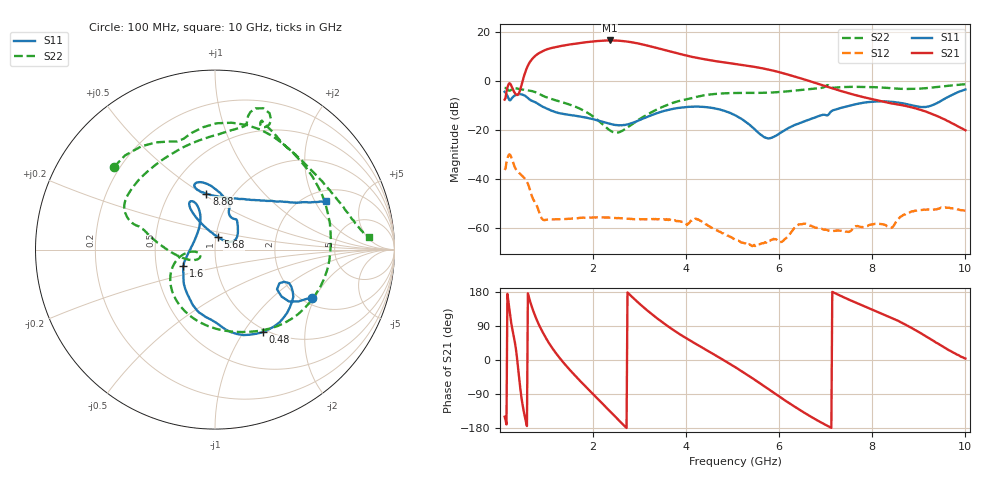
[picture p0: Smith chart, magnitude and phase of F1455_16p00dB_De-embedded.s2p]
! Integrated Device Technology
! Corporate Headquarters
! 6024 Silver Creek Valley Road
! San Jose, CA 95138  USA
! Phone:  1-408-284-8200
! Toll Free:  1-800-223-1366
! Webpage:  http://www.idt.com/
! Timing and RF Division
! 515 Groton Road, Suite 102
! Westford, MA 01886-6024
! Device:  F1455
! Description: 6-bit 0.5 dB Transmit Variable Gain Amplifier
! Frequency:  1400.0 -  2300.00 MHz
! Package:  6x6 mm Thin QFN Plastic Package: 28 pin
! State:  32
! Atten State:  16.0 dB
! Voltage:  +5.00 Volts
! Current:  217.655 mA
! Data:  The device was measured on a the F1455 evaluation board which has
!  individual transmission lines to the RF pins.  Data was collected
!  using a calibrated network analyzer.  The evaluation board was
!  de-embedded using a TRL calibration technique.
!  The reference plane is the edge of the package pin.
!  Pin  1 = CSb
!  Pin  2 = DATA
!  Pin  3 = CLK
!  Pin  4 = RSET
!  Pin  5 = GND
!  Pin  6 = RFIN  = Port 1
!  Pin  7 = GND
!  Pin  8 = NC
!  Pin  9 = NC
!  Pin 10 = NC
!  Pin 11 = NC
!  Pin 12 = NC
!  Pin 13 = NC
!  Pin 14 = /STBY
!  Pin 15 = GND
!  Pin 16 = RFOUT  = Port 2
!  Pin 17 = GND
!  Pin 18 = NC
!  Pin 19 = NC
!  Pin 20 = NC
!  Pin 21 = GND
!  Pin 22 = NC
!  Pin 23 = GND
!  Pin 24 = NC
!  Pin 25 = NC
!  Pin 26 = NC
!  Pin 27 = GND
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# GHz S dB R 50
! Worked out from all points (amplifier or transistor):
!   496 points, 100 MHz to 10 GHz, reference 50 ohm
!   highest |S21| = 16.6 dB at 2.36 GHz (marker M1)
!   |S21| within 3 dB of that: 1.129 GHz to 3.356 GHz (2.227 GHz wide, 99.3 % of centre)
!   unconditionally stable (mu >= 1): start of sweep to end of sweep
!   at 1.74 GHz: K = 45.78, MAG = 16.1 dB, |S12| = -55.8 dB
!   at 5.06 GHz: K = 250.94, MAG = 8.9 dB, |S12| = -64.8 dB
!   at 10 GHz: K = 311.19, MAG = -11.5 dB, |S12| = -52.9 dB
!   S11 on the Smith chart (normalised r, x): 100 MHz: 2.25, -1.91; 480 MHz: 0.96, -1.23; 1.6 GHz: 0.69, -0.13; 5.68 GHz: 1.02, +0.14; 8.88 GHz: 0.75, +0.52; 10 GHz: 2.48, +2.47
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0.1  -4.35 -26.3  -7.54 -149.7  -36.29 46.5  -2.77 140.7
0.26  -6.85 -24.3  -2.57 85.2  -32.06 -76.5  -3.29 95.6
0.48  -5.48 -59.8  -0.37 -113.8  -38.74 -146.9  -3.44 31.8
0.68  -7.99 -91.2  8.77 142.1  -46.65 142.8  -4.02 -14.9
0.8  -9.07 -106.7  10.96 103.2  -51.22 123.4  -4.81 -42.1
0.94  -10.65 -121.4  12.45 68.5  -56.75 123.4  -6.14 -68.4
1.26  -13.00 -142.0  14.17 8.9  -56.46 97.2  -8.17 -112.3
1.6  -14.07 -152.8  15.27 -39.3  -56.09 67.2  -10.30 -144.6
1.76  -14.57 -157.1  15.69 -60.0  -55.81 55.8  -11.64 -156.3
2.06  -15.84 -166.7  16.33 -97.4  -55.72 37.6  -15.28 -172.1
2.36  -17.45 175.8  16.62 -134.9  -55.79 22.2  -20.09 -170.6
2.56  -18.03 157.9  16.51 -159.8  -55.97 13.7  -20.89 -155.2
2.76  -17.61 139.1  16.10 175.8  -56.25 7.1  -18.66 -151.4
3.08  -15.26 118.8  14.92 139.6  -56.43 -2.4  -14.58 -165.8
3.4  -12.91 112.1  13.40 107.8  -56.41 -12.3  -11.35 179.3
4.08  -10.49 115.6  10.11 51.7  -57.61 -26.8  -7.12 163.1
5.06  -14.00 120.1  7.00 -19.3  -64.83 -68.6  -4.83 148.0
5.68  -22.94 78.0  5.08 -69.3  -66.06 -44.8  -4.76 123.0
6.7  -15.33 41.8  -0.28 -151.0  -59.23 -130.8  -3.18 78.4
8.36  -8.35 107.1  -8.90 113.7  -59.78 141.2  -2.82 62.4
8.88  -10.04 98.8  -10.91 82.1  -53.27 136.0  -3.18 41.9
10  -3.42 23.7  -20.07 3.8  -52.93 55.2  -1.29 4.6
